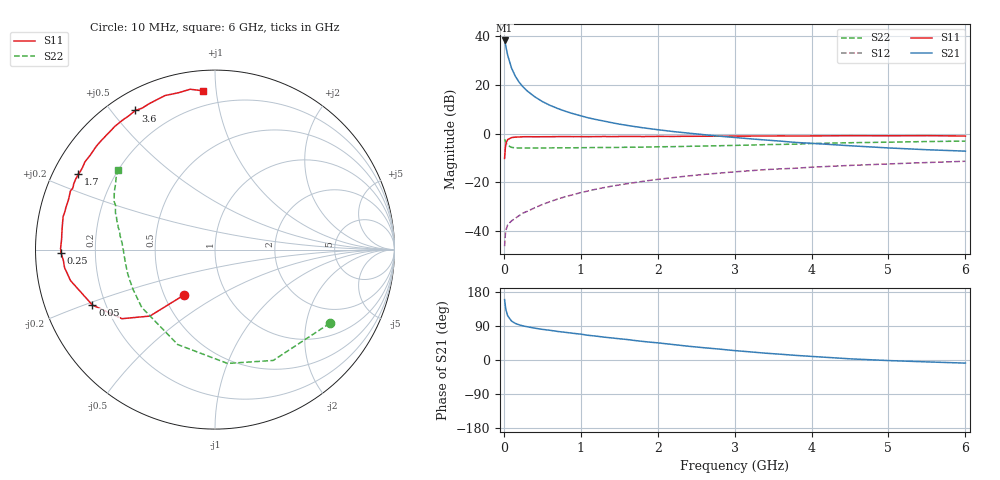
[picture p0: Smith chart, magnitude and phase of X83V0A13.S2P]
! SIEMENS Small Signal Semiconductors
! BFP136W
! Si NPN RF Bipolar Junction Transistor in SOT343
! VCE = 3 V  IC = 130 mA
! Common Emitter S-Parameters:  September  1994
# GHz  S  MA  R  50
!  f  S11  S21  S12  S22
! GHz  MAG  ANG  MAG  ANG  MAG  ANG  MAG  ANG
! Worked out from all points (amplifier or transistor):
!   40 points, 10 MHz to 6 GHz, reference 50 ohm
!   highest |S21| = 38.2 dB at 10 MHz (marker M1)
!   |S21| within 3 dB of that: start of sweep to 29.73 MHz
!   unconditionally stable (mu >= 1): 462.9 MHz to 2.969 GHz
!   at 200 MHz: K = 0.74, MSG = 27.3 dB, |S12| = -33.6 dB
!   at 1.5 GHz: K = 1.10, MAG = 10.6 dB, |S12| = -21.1 dB
!   at 6 GHz: K = 0.98, MSG = 2.1 dB, |S12| = -11.4 dB
!   S11 on the Smith chart (normalised r, x): 10 MHz: 0.63, -0.35; 50 MHz: 0.15, -0.21; 250 MHz: 0.08, -0.01; 1.7 GHz: 0.07, +0.26; 3.6 GHz: 0.08, +0.58; 6 GHz: 0.11, +0.92
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0.01  0.3087 -124.5  80.85 159.3  0.0049 66.6  0.7602 -32.7
0.02  0.5183 -134.4  68.64 142.2  0.0087 54.8  0.6975 -62.3
0.03  0.6456 -143.4  56.95 130.4  0.0108 48.2  0.6381 -83.7
0.05  0.7498 -155.7  40.11 116.6  0.0134 39.8  0.5684 -111.4
0.1  0.8234 -167.9  21.95 102.7  0.0162 38.7  0.52 -141.7
0.15  0.8443 -173.2  14.89 96.5  0.0183 42.5  0.5075 -153.9
0.2  0.8473 -176.0  11.19 92.7  0.0208 44.7  0.5046 -160.4
0.25  0.8576 -178.6  9.027 90.0  0.0234 47.5  0.5045 -164.6
0.3  0.8605 179.6  7.546 87.9  0.0252 50.6  0.5038 -167.4
0.4  0.8566 176.3  5.682 84.1  0.0299 54.2  0.5047 -171.3
0.5  0.8583 173.8  4.53 80.9  0.035 56.9  0.5052 -173.9
0.6  0.86 171.9  3.778 78.4  0.0401 59.0  0.5066 -175.6
0.7  0.8635 169.2  3.258 75.3  0.0453 60.8  0.5081 -176.9
0.9  0.8627 165.8  2.551 70.5  0.0557 61.7  0.5098 -179.4
1.1  0.8621 161.5  2.089 65.1  0.0666 61.9  0.5133 178.9
1.7  0.8697 151.0  1.389 51.5  0.0986 59.6  0.5244 174.0
2.2  0.8719 142.8  1.098 40.8  0.1247 55.6  0.5376 170.3
3.2  0.8863 125.8  0.779 21.5  0.1724 45.8  0.5794 161.4
3.6  0.8931 119.8  0.697 15.2  0.1884 41.9  0.5985 158.0
4.5  0.9024 108.0  0.561 3.1  0.2217 33.4  0.647 150.1
5.5  0.9042 98.8  0.465 -5.0  0.2539 25.5  0.6844 143.5
6  0.8873 94.4  0.435 -8.2  0.2699 21.1  0.6986 140.6
